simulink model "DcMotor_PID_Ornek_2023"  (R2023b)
settings: Solver=VariableStepAuto  StartTime=0.0  StopTime=10.0  RelTol=1e-3
libraries: fl_lib x5, nesl_utility x4, ee_lib x1, simulink x1, slpidlib x1

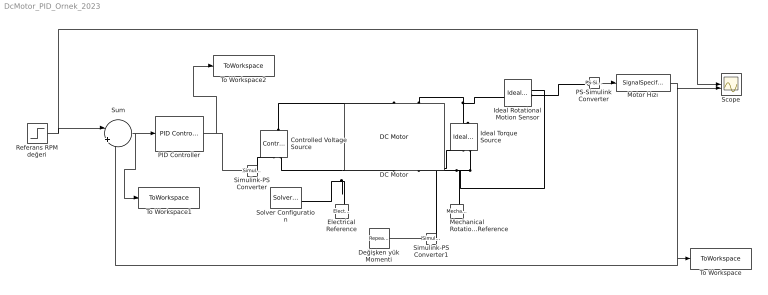
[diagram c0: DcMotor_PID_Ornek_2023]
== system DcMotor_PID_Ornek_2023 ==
  Controlled Voltage Source : fl_lib/Electrical/Electrical Sources/Controlled Voltage Source
  DC Motor : ee_lib/Electromechanical/Brushed Motors/DC Motor  Tag={'toolbox/physmod/elec/library/m/ee_lib_parts';'Electromechanical/Brushed_Motors/DC_Motor/Crouzet/x89_850_007.xml'}  field_option=ee.enum.field_option.pm  Rf=100 % Parameter not set Ohm  Lf=1 % Parameter not set H  Laf=0.15 % Parameter not set H  If0=0 % Parameter not set A  parameterization=ee.enum.dcparam_option.load_speed  Ra=0.8 Ohm  La=0.5 mH  emf_or_torque=ee.enum.emf_or_torque.kv  Kv=3.04 mV/rpm  Ki=29.02986 % Parameter estimated mN*m/A  T_stall=0.24e-3 % Parameter not set N*m  w_max=4000 rpm  w_rated=3000 rpm  P_rated=50 W  V_rated=12 V  lam_param=ee.enum.lam_param.current  i_noload=0.31 A  V_i_noload=12 V  J=160 g*cm^2  lam=0 % % Parameter not set mN*m/(rad/s)  speed0=0 % Parameter not set rpm  t_fault_armature=1 % Parameter not set s  t_fault_field=1 % Parameter not set s  fault_action=simscape.enum.assert.action.none  alpha=3.93e-3 % Parameter not set 1/K  Tmeas=25 % Parameter not set degC  thermal_mass=124 % Parameter assumed J/K  initial_temperature=25 % Parameter not set degC
  Değişken yük Momenti : simulink/Sources/Repeating Sequence Stair  OutValues=[0.2 -0.2 -0.2 -0.32 -0.3].'  tsamp=1  OutMin=[]  OutMax=[]  OutDataTypeStr=double  OutputDataTypeScalingMode=double  OutDataType=fixdt(0,8)  ConRadixGroup=Best Precision: Vector-wise  OutScaling=2^-12
  Electrical Reference : fl_lib/Electrical/Electrical Elements/Electrical Reference
  Ideal Rotational Motion Sensor : fl_lib/Mechanical/Mechanical Sensors/Ideal Rotational Motion Sensor  reference=foundation.enum.MeasurementReference.difference  acceleration_port=false  velocity_port=true  position_port=true  wrap_angle=false  offset=0 rad
  Ideal Torque Source : fl_lib/Mechanical/Mechanical Sources/Ideal Torque Source
  Mechanical Rotational Reference : fl_lib/Mechanical/Rotational Elements/Mechanical Rotational Reference
  Motor Hızı : SignalSpecification  Unit=rpm
  PID Controller : slpidlib/PID Controller  Controller=PID  Form=Parallel  TimeDomain=Continuous-time  UseExternalTs=off  SampleTime=-1  IntegratorMethod=Forward Euler  FilterMethod=Forward Euler  ControllerParametersSource=internal  P=0.00475587671986985  I=0.806268943220032  UseKiTs=off  D=2.16390412417395e-06  N=21175.469508566  UseFilter=on  TunerSelectOption=Transfer Function Based (PID Tuner App)  InitialConditionSource=internal  InitialConditionForIntegrator=0  InitialConditionForFilter=0  DifferentiatorICPrevScaledInput=0  ExternalReset=none  TrackingMode=off  Kt=1  LimitOutput=on  SatLimitsSource=internal  UpperSaturationLimit=15  LowerSaturationLimit=0  LinearizeAsGain=on  AntiWindupMode=none  Kb=1  LimitIntegrator=off  UpperIntegratorSaturationLimit=inf  LowerIntegratorSaturationLimit=-inf  POutMin=[]  POutMax=[]  IOutMin=[]  IOutMax=[]  DOutMin=[]  DOutMax=[]  NOutMin=[]  NOutMax=[]  SumOutMin=[]  SumOutMax=[]  SaturationOutMin=[]  SaturationOutMax=[]  PParamMin=[]  PParamMax=[]  IParamMin=[]  IParamMax=[]  DParamMin=[]  DParamMax=[]  NParamMin=[]  NParamMax=[]  KbParamMin=[]  KbParamMax=[]  KtParamMin=[]  KtParamMax=[]  KbOutMin=[]  KbOutMax=[]  KtOutMin=[]  KtOutMax=[]  IntegratorOutMin=[]  IntegratorOutMax=[]  FilterOutMin=[]  FilterOutMax=[]  SumI1OutMin=[]  SumI1OutMax=[]  SumI2OutMin=[]  SumI2OutMax=[]  SumI3OutMin=[]  SumI3OutMax=[]  SumI4OutMin=[]  SumI4OutMax=[]  SumDOutMin=[]  SumDOutMax=[]  DifferentiatorOutMin=[]  DifferentiatorOutMax=[]  FilterDiffOutCoefMin=[]  FilterDiffOutCoefMax=[]  ReciprocalOutMin=[]  ReciprocalOutMax=[]  SumDenOutMin=[]  SumDenOutMax=[]  SumNumOutMin=[]  SumNumOutMax=[]  DivideOutMin=[]  DivideOutMax=[]  UdiffTsProdOutMin=[]  UdiffTsProdOutMax=[]  NTsProdOutMin=[]  NTsProdOutMax=[]  UintegralTsProdOutMin=[]  UintegralTsProdOutMax=[]  UngainTsProdOutMin=[]  UngainTsProdOutMax=[]  ClampingZeroOutDataTypeStr=Inherit: Inherit via back propagation  ClampingZeroOutMin=[]  ClampingZeroOutMax=[]  FilterDenConstantOutDataTypeStr=Inherit: Inherit via back propagation  FilterDenConstantOutMin=[]  FilterDenConstantOutMax=[]  PCopyOutDataTypeStr=Inherit: Inherit via back propagation  PCopyOutMin=[]  PCopyOutMax=[]  NCopyOutDataTypeStr=Inherit: Inherit via back propagation  NCopyOutMin=[]  NCopyOutMax=[]  IntegratorContinuousStateAttributes=''  IntegratorStateMustResolveToSignalObject=off  IntegratorRTWStateStorageClass=Auto  FilterContinuousStateAttributes=''  FilterStateMustResolveToSignalObject=off  FilterRTWStateStorageClass=Auto  ParallelPVariant=InternalParameters  IdealPVariant=Disabled  IVariant=InternalParameters  DVariant=InternalParameters  IntegratorVariant=Continuous  SatVariant=Enabled  AWVariant=Passthrough  PCopyVariant=Disabled  TRVariant=Disabled  FdbkBlocksVariant=Forward  IdealPFdbkVariant=Disabled  SatFdbkVariant=Disabled  DerivativeFilterVariant=ContFilter  NVariant=InternalParameters  NCopyVariant=Disabled  FilterICVariant=InternalICsFilter  IntegratorICVariant=InternalICs  ExternalResetVariant=Disabled  TRSumVariant=Passthrough  SumFdbkVariant=Disabled  SumVariant=Sum_PID  TsampFilterVariant=InternalTs  TsampNgainVariant=Passthrough  TsampIntegralVariant=Disabled_SignalSpec  ExternalSaturationOutDataTypeStr=Inherit: Same as second input
  PS-Simulink Converter : nesl_utility/PS-Simulink Converter  PhysicalDomain=network_engine_domain  SubClassName=ps_output  LeftPortType=input  RightPortType=output  PseudoPeriodic=off  Frequencies=[]  VectorFormat=inherit  Unit=inherit  AffineConversion=off
  Referans RPM değeri : Step  Time=0  After=2500  SampleTime=0
  Scope : Scope  NumInputPorts=2
  Simulink-PS Converter : nesl_utility/Simulink-PS Converter  PhysicalDomain=network_engine_domain  SubClassName=ps_input  LeftPortType=input  RightPortType=output  PseudoPeriodic=off  Frequencies=[]  NoiseDistribution=none  NoiseParameters=[]  Unit=1  AffineConversion=off  FilteringAndDerivatives=provide  SimscapeFilterOrder=1  InputFilterTimeConstant=0.001  UdotUserProvided=0
  Simulink-PS Converter1 : nesl_utility/Simulink-PS Converter  PhysicalDomain=network_engine_domain  SubClassName=ps_input  LeftPortType=input  RightPortType=output  PseudoPeriodic=off  Frequencies=[]  NoiseDistribution=none  NoiseParameters=[]  Unit=1  AffineConversion=off  FilteringAndDerivatives=provide  SimscapeFilterOrder=1  InputFilterTimeConstant=0.001  UdotUserProvided=0
  Solver Configuration : nesl_utility/Solver Configuration  PhysicalDomain=network_engine_domain  SubClassName=solver  LeftPortType=input  RightPortType=generic  Tones=[]  Harmonics=[]  SimulateNoise=off  Profile=off  UseLocalSampling=off  EnableSwitchedLinearOptims=on  FrequencyDomain=off  UseCCode=off  RelTol=0.001  AbsTol=0.001  MinStep=1e-09  ToWorkspace=off  RevertToSquareIcSolve=off  NumHomotopyIterations=100  PhasorMode=off  PhasorModeNumHarmonics=1  ConsistencySolver=NEWTON_XTOL_AFTER_FTOL  IndexReductionMethod=DerivativeReplacement  DoDC=off  ResidualTolerance=1e-09  ConsistencyTolSource=GLOBAL  ConsistencyAbsTol=0.001  ConsistencyRelTol=0.001  ConsistencyTolFactor=0.001  UseLocalSolver=off  LocalSolverChoice=NE_BACKWARD_EULER_ADVANCER  ResolveIndetEquations=on  FunctionEvalNumThread=1  LocalSolverSampleTime=0.001  DoFixedCost=off  MaxNonlinIter=3  MaxModeIter=2  ComputeImpulses=off  ImpulseIterations=2  LinearAlgebra=auto  LinearAlgebraNumThread=0  EquationFormulation=NE_TIME_EF  DelaysMemoryBudget=1024  AutomaticFiltering=on  FilteringTimeConstant=0.001  PartitionStorageMethod=AS_NEEDED  PartitionMemoryBudget=1024  PartitionMethod=ROBUST  MultibodyUseLocalSolver=off  MultibodyLocalSolverChoice=ODE1  MultibodyLocalSolverSampleTime=0.001
  Sum : Sum  Inputs=|+-
  To Workspace : ToWorkspace  VariableName=RPM_Hiz  SaveFormat=Timeseries  SampleTime=-1
  To Workspace1 : ToWorkspace  VariableName=Hata  SaveFormat=Timeseries  SampleTime=-1
  To Workspace2 : ToWorkspace  VariableName=PID_Cikis  SaveFormat=Timeseries  SampleTime=-1
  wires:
  PS-Simulink Converter/1 -> Motor Hızı/1
  Motor Hızı/1 -> Scope/2, Sum/2, To Workspace/1
  Değişken yük Momenti/1 -> Simulink-PS Converter1/1
  Referans RPM değeri/1 -> Scope/1, Sum/1
  Sum/1 -> To Workspace1/1, PID Controller/1
  PID Controller/1 -> To Workspace2/1, Simulink-PS Converter/1
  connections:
  Controlled Voltage Source/LConn1 -- DC Motor/LConn1
  Controlled Voltage Source/RConn2 -- Solver Configuration/RConn1 -- Electrical Reference/LConn1 -- DC Motor/RConn1
  Simulink-PS Converter/RConn1 -- Controlled Voltage Source/RConn1
  Ideal Rotational Motion Sensor/RConn2 -- PS-Simulink Converter/LConn1
  DC Motor/LConn2 -- Ideal Rotational Motion Sensor/LConn1 -- Ideal Torque Source/LConn1
  Ideal Torque Source/RConn2 -- Mechanical Rotational Reference/LConn1 -- DC Motor/RConn2 -- Ideal Rotational Motion Sensor/RConn1
  Simulink-PS Converter1/RConn1 -- Ideal Torque Source/RConn1
